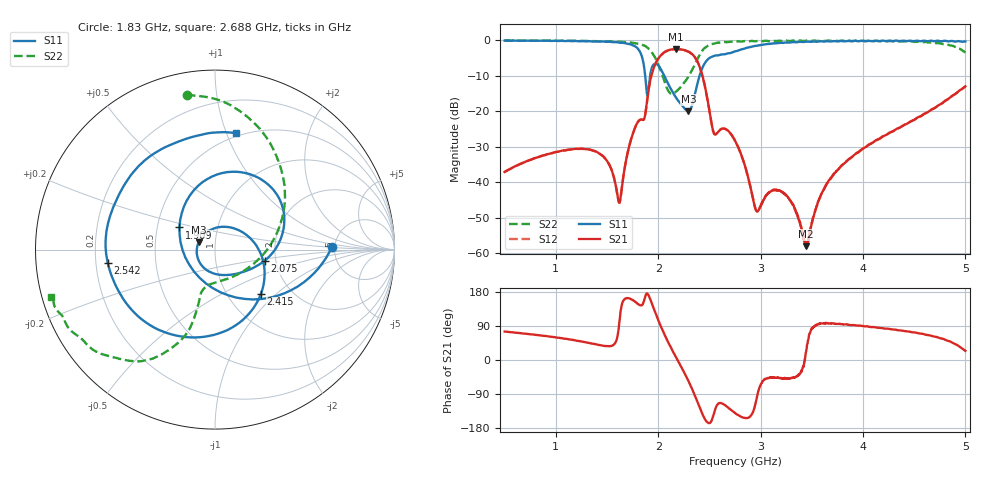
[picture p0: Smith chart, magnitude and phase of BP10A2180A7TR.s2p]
!Agilent Technologies,E8358A,US41080443,A.07.50.56
!Agilent E8358A: A.07.50.56
!Date: Tuesday, December 16, 2014 13:47:42
!Correction: S11(Full 2 Port(1,2))
!S21(Full 2 Port(1,2))
!S12(Full 2 Port(1,2))
!S22(Full 2 Port(1,2))
!S2P File: Measurements: S11, S21, S12, S22:
# Hz S  dB  R 50
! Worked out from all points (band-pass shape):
!   1601 points, 500 MHz to 5 GHz, reference 50 ohm
!   highest |S21| = -2.46 dB at 2.173 GHz (marker M1); lowest = -58.1 dB at 3.442 GHz (marker M2)
!   |S21| within 3 dB of the highest: 1.994 GHz to 2.373 GHz (379.5 MHz wide, 17.4 % of centre)
!   lowest |S11| = -20.0 dB at 2.294 GHz (marker M3), VSWR 1.22, Z = 41.5 + j3.36 ohm
!   |S11| at or under -10 dB: 1.873 GHz to 1.921 GHz (47.65 MHz wide, 2.51 % of centre); 2.059 GHz to 2.404 GHz (344.5 MHz wide, 15.4 % of centre)
!   |S22| runs from -15.1 to 0.0 dB; largest |S21 - S12| = 0.0033
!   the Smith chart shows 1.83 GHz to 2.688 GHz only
!   S11 on the Smith chart (normalised r, x): 1.83 GHz: 4.72, +0.25; 1.909 GHz: 0.65, +0.17; 2.075 GHz: 1.74, -0.23; 2.415 GHz: 1.42, -0.81; 2.542 GHz: 0.25, -0.06; 2.688 GHz: 0.47, +1.08
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5e8  -0.08 161.9  -37.13 75.1  -37.15 75.1  -0.05 171.9
1.250938e9  -0.20 125.0  -30.59 48.8  -30.62 49.0  -0.15 153.0
1.619375e9  -0.65 83.0  -45.79 96.3  -45.83 96.9  -0.39 131.2
1.830312e9  -3.72 1.3  -22.32 144.0  -22.36 143.7  -1.15 100.4
1.909062e9  -12.63 148.1  -13.37 169.0  -13.40 169.2  -2.42 75.6
2.001875e9  -7.11 30.5  -5.10 104.2  -5.11 104.2  -6.81 32.0
2.075e9  -10.96 -12.6  -3.09 59.4  -3.11 59.4  -12.78 -20.0
2.173438e9  -16.13 -65.2  -2.46 7.6  -2.47 7.6  -14.48 -93.9
2.294375e9  -20.01 156.3  -3.17 -54.8  -3.19 -54.7  -10.24 -107.0
2.415312e9  -8.97 -44.3  -8.39 -132.5  -8.40 -132.4  -3.62 -117.2
2.541875e9  -4.40 -172.9  -26.03 -143.1  -26.09 -143.2  -0.95 -146.7
2.688125e9  -3.62 79.6  -25.66 -126.8  -25.69 -126.3  -0.45 -164.0
2.75e9  -3.11 42.7  -28.26 -140.2  -28.32 -139.7  -0.40 -169.2
2.955312e9  -1.55 -38.2  -47.92 -108.9  -47.97 -109.1  -0.23 179.0
3.045312e9  -1.11 -59.1  -44.06 -50.5  -44.16 -50.9  -0.12 175.2
3.250625e9  -0.60 -91.2  -43.75 -48.7  -43.86 -49.0  -0.07 168.3
3.441875e9  -0.36 -109.2  -58.06 20.2  -58.07 16.0  -0.10 163.1
3.500938e9  -0.34 -113.6  -51.54 82.0  -51.64 80.3  -0.15 161.7
3.723125e9  -0.21 -128.0  -37.40 96.1  -37.40 95.9  -0.06 156.5
4.251875e9  -0.08 -149.8  -26.18 82.3  -26.23 82.3  -0.24 143.3
4.727188e9  -0.09 -165.4  -18.49 60.1  -18.52 60.2  -0.77 117.7
5e9  -0.29 -172.5  -12.97 24.0  -13.00 23.8  -3.45 57.9
